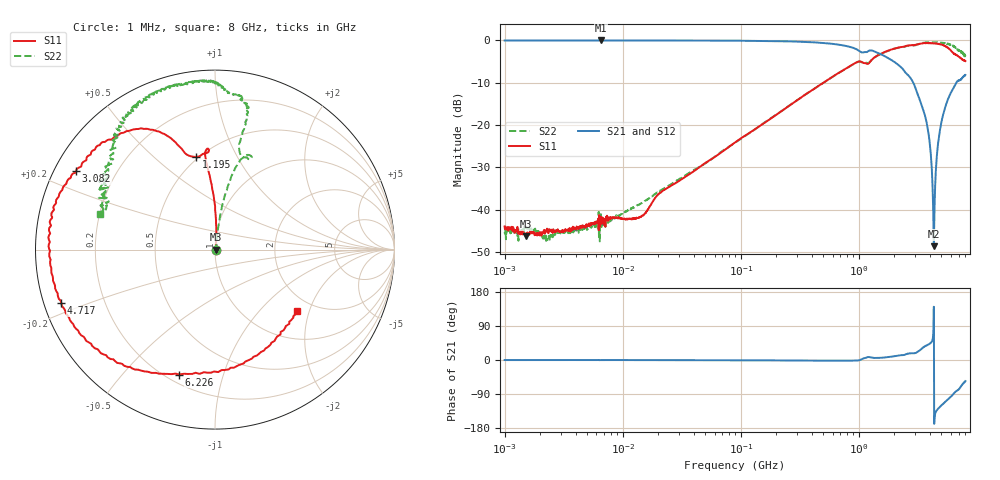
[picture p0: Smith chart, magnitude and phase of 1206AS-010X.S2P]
!s-Parameter Generated by FASTRON Sdn. Bhd.
!FASTRON P/N : 1206AS-010X
!Keysight Technologies: E5071C_MY46733604_B.14.02
!Date: Wed Nov 15 09:35:17 2023
!Version  :Rev00  Wed Nov 15 09:35:17 2023
!Data & Calibration Information:
!Freq  S11:SOLT2(ON)  S21:SOLT2(ON)  S12:SOLT2(ON)  S22:SOLT2(ON)
!PortZ  Port1:50+j0  Port2:50+j0
!When reading reference impedance value at option line is always used.
! Remarks : This data is being provided solely for informational purposes.
# Hz S dB R 50
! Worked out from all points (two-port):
!   1601 points, 1 MHz to 8 GHz, reference 50 ohm
!   highest |S21| = -0.04 dB at 6.499 MHz (marker M1); lowest = -48.6 dB at 4.325 GHz (marker M2)
!   |S21| within 3 dB of the highest: start of sweep to 1.466 GHz
!   lowest |S11| = -46.2 dB at 1.505 MHz (marker M3), VSWR 1.01, Z = 50.5 - j0.107 ohm
!   |S11| at or under -10 dB: start of sweep to 504.4 MHz
!   |S22| runs from -47.5 to -0.5 dB; largest |S21 - S12| = 0.0063
!   S11 on the Smith chart (normalised r, x): 1 MHz: 1.01, -0.00; 1.195 GHz: 0.49, +0.70; 3.082 GHz: 0.06, +0.26; 4.717 GHz: 0.05, -0.17; 6.226 GHz: 0.25, -0.72; 8 GHz: 1.65, -1.66
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1000000  -43.93 -15.1  -0.05 -0.2  -0.06 -0.1  -45.29 -14.5
1504644  -46.23 -12.5  -0.04 -0.1  -0.05 -0.0  -44.77 -22.2
2311589  -44.88 12.2  -0.05 -0.1  -0.06 -0.1  -47.16 21.6
4479405  -43.85 27.4  -0.05 -0.1  -0.06 -0.1  -44.69 30.6
6498814  -41.61 34.9  -0.04 -0.2  -0.07 -0.1  -43.27 19.0
1.406113e7  -41.67 63.5  -0.05 -0.2  -0.06 -0.2  -38.67 52.6
2.00676e7  -36.32 66.6  -0.05 -0.2  -0.07 -0.1  -35.79 66.3
8.994653e7  -24.04 83.2  -0.09 -0.6  -0.10 -0.6  -24.14 80.7
4.006501e8  -11.81 90.4  -0.45 -1.6  -0.45 -1.6  -11.82 80.6
9.405027e8  -5.30 95.8  -2.02 -1.7  -2.03 -1.8  -5.34 72.6
1.19487e9  -5.56 101.3  -2.62 7.8  -2.63 7.7  -5.36 72.7
1.7949e9  -2.41 118.2  -4.28 7.9  -4.29 7.7  -2.43 76.7
3.08186e9  -1.02 150.6  -12.03 19.7  -12.05 19.6  -1.05 85.7
3.811538e9  -0.59 170.5  -20.35 39.8  -20.35 39.7  -0.48 94.0
4.034495e9  -0.71 177.2  -25.50 44.6  -25.47 44.5  -0.52 97.3
4.196646e9  -0.69 -177.7  -33.02 51.6  -33.00 51.5  -0.52 97.8
4.324643e9  -0.75 -173.6  -48.59 140.5  -48.68 140.3  -0.49 101.3
4.492594e9  -0.77 -168.1  -30.91 -137.7  -30.90 -137.8  -0.55 102.1
4.716529e9  -0.85 -160.8  -23.94 -128.1  -23.90 -128.2  -0.50 106.3
5.276366e9  -1.21 -142.0  -16.70 -113.4  -16.67 -113.6  -0.70 115.5
6.226476e9  -2.80 -106.0  -11.67 -92.3  -11.65 -92.7  -1.29 127.3
8e9  -4.89 -36.6  -8.18 -55.7  -8.16 -56.3  -3.47 162.9
